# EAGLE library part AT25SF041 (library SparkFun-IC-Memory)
AT25SF041 4Mb Serial Flash Memory 104MHz, SPI, 8-SOIC Datasheet SparkFun Products: SparkFun ESP8266 Thing SparkFun ESP8266 Thing - Dev Board
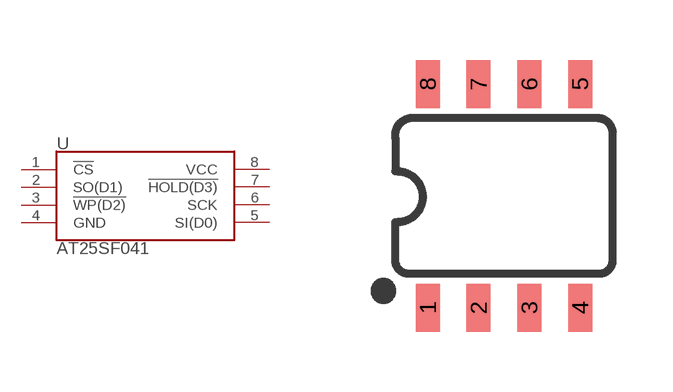
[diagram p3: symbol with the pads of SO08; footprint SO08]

Designator prefix U

## AT25SF041 (PROD_ID: IC-12455; VALUE: 4MB Flash)  [SO08]
1  !CS
2  SO(D1)
3  !WP(D2)
4  GND
5  SI(D0)
6  SCK
7  !HOLD(D3)
8  VCC

## Footprint SO08 (pad centres in mm)
SOIC, 0.15 inch width
smd 0.6 x 1.2: 1 -1.905,-2.8; 2 -0.635,-2.8; 3 0.635,-2.8; 4 1.905,-2.8; 5 1.905,2.8; 6 0.635,2.8; 7 -0.635,2.8; 8 -1.905,2.8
